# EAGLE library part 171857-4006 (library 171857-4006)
Headers & Wire Housings KK RPC 254 Hdr FrLk R/A 06 Ckt 15Au T&R Source: Datasheet
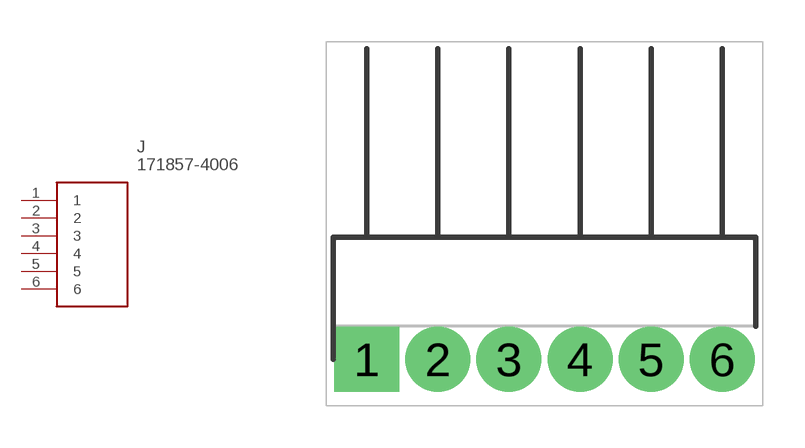
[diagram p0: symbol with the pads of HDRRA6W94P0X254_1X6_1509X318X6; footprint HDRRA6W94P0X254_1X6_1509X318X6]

Designator prefix J

## 171857-4006 (Description: Headers & Wire Housings KK RPC 254 Hdr FrLk R/A 06 Ckt 15Au T&R; Height: 6.35mm; Manufacturer_Name: Molex; Manufacturer_Part_Number: 171857-4006; Mouser_Part_Number: 538-171857-4006; Mouser_Price-Stock: https://www.mouser.co.uk/ProductDetail/Molex/171857-4006?qs=v0t%252BUMfTP8OU%2F3VfGCmihQ%3D%3D)  [HDRRA6W94P0X254_1X6_1509X318X6]
1  1
2  2
3  3
4  4
5  5
6  6

## Footprint HDRRA6W94P0X254_1X6_1509X318X6 (pad centres in mm)
171857-4006
drill 1.55 pad 2.325 square: 1 0,0
drill 1.55 pad 2.325: 2 2.54,0; 3 5.08,0; 4 7.62,0; 5 10.16,0; 6 12.7,0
